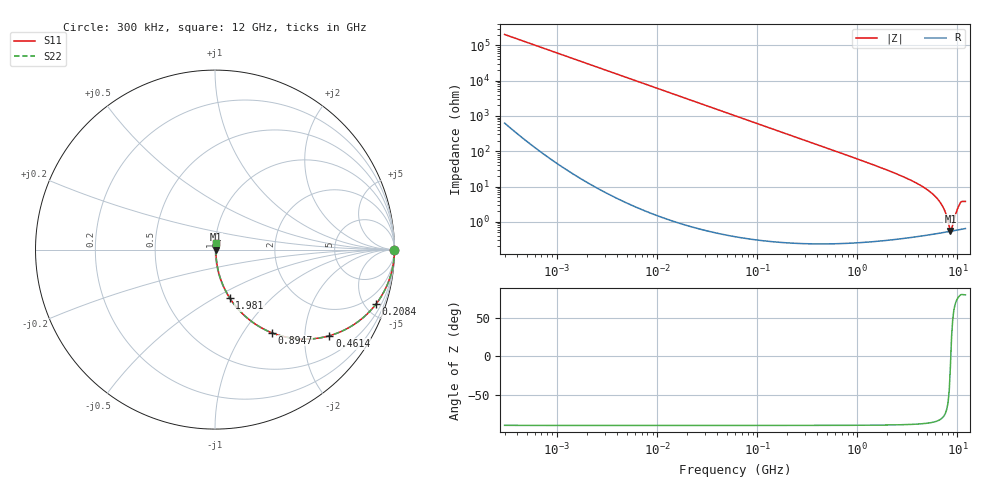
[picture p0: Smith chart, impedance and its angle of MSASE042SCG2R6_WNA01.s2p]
! MSASE042SCG2R6_WNA01  S-PARAMETER MODEL  ( General Type )
! Model Generated by TAIYO YUDEN Corporation (http://www.ty-top.com)
! Version 1.0
! TAIYO YUDEN Control No. 130801
! Copyright(c) 2013 TAIYO YUDEN CO.,LTD. All Rights Reserved.
! Product Description (link to TY-COMPAS)
! https://ds.yuden.co.jp/TYCOMPAS/or/detail?pn=MSASE042SCG2R6AWNA01&u=M
! Products Name : Multilayer Ceramic Capacitors
! Characteristics :
!  Capacitance : 2.6 pF , Rated Voltage : 16V , TCC : CG / C0G
!  Case Size : 0.4 x 0.2 / 0.016 x 0.008 [mm/inch] , Thickness : 0.2 / 0.008 [mm/inch]
!  (Conditions: Temperature = 25 degC , DC Bias Current/Voltage = 0A / 0V)
! External Node Assignments :
!  1  o---| |---o  2
! GND o---------o GND
! Frequency Range : 0.3MHz  -  12000MHz  [ 401 STEP ]
# MHz S RI R 50
! Freq[MHz].  S11 Real  S11 Imag  S21 Real  S21 Imag  S12 Real  S12 Imag  S22 Real  S22 Imag
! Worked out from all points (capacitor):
!   401 points, 300 kHz to 12 GHz, reference 50 ohm
!   read as one part in series: C = 2.6 pF near 316.3 kHz
!   lowest |Z| = 551 mohm at 8.504 GHz (marker M1)
!   series resonance near 8.577 GHz, so ESL is about 130 pH
!   S11 on the Smith chart (normalised r, x): 300 kHz: open; 208.4 MHz: 1.01, -5.88; 461.4 MHz: 1.00, -2.65; 894.7 MHz: 1.00, -1.36; 1.981 GHz: 1.01, -0.59; 12 GHz: 1.01, +0.07
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0.3  1 -0.000489  1.74e-06 0.000489  1.74e-06 0.000489  1 -0.000489
1.769972  1 -0.00289  9.66e-06 0.00289  9.66e-06 0.00289  1 -0.00289
10.44266  0.9997 -0.017  0.000294 0.017  0.000294 0.017  0.9997 -0.017
60  0.9905 -0.0969  0.00952 0.0969  0.00952 0.0969  0.9905 -0.0969
208.3979  0.8962 -0.3046  0.1038 0.3046  0.1038 0.3046  0.8962 -0.3046
353.9943  0.7491 -0.4328  0.2509 0.4328  0.2509 0.4328  0.7491 -0.4328
461.3684  0.637 -0.48  0.363 0.48  0.363 0.48  0.637 -0.48
894.6982  0.3155 -0.4629  0.6845 0.4629  0.6845 0.4629  0.3155 -0.4629
1331.232  0.1696 -0.3723  0.8304 0.3723  0.8304 0.3723  0.1696 -0.3723
1980.756  0.0814 -0.2684  0.9186 0.2684  0.9186 0.2684  0.0814 -0.2684
2088.533  0.0733 -0.2552  0.9267 0.2552  0.9267 0.2552  0.0733 -0.2552
3841.137  0.0196 -0.1247  0.9804 0.1247  0.9804 0.1247  0.0196 -0.1247
5715.274  0.00792 -0.059  0.9921 0.059  0.9921 0.059  0.00792 -0.059
7064.448  0.00565 -0.0277  0.9944 0.0277  0.9944 0.0277  0.00565 -0.0277
7648.807  0.00534 -0.0163  0.9947 0.0163  0.9947 0.0163  0.00534 -0.0163
8281.503  0.0053 -0.00505  0.9947 0.00505  0.9947 0.00505  0.0053 -0.00505
8503.825  0.00534 -0.00121  0.9947 0.00121  0.9947 0.00121  0.00534 -0.00121
8966.534  0.00553 0.00606  0.9945 -0.00606  0.9945 -0.00606  0.00553 0.00606
9708.23  0.00602 0.0173  0.994 -0.0173  0.994 -0.0173  0.00602 0.0173
10511.28  0.0069 0.0306  0.9931 -0.0306  0.9931 -0.0306  0.0069 0.0306
11083.22  0.00748 0.0367  0.9925 -0.0367  0.9925 -0.0367  0.00748 0.0367
12000  0.00775 0.0366  0.9922 -0.0366  0.9922 -0.0366  0.00775 0.0366
